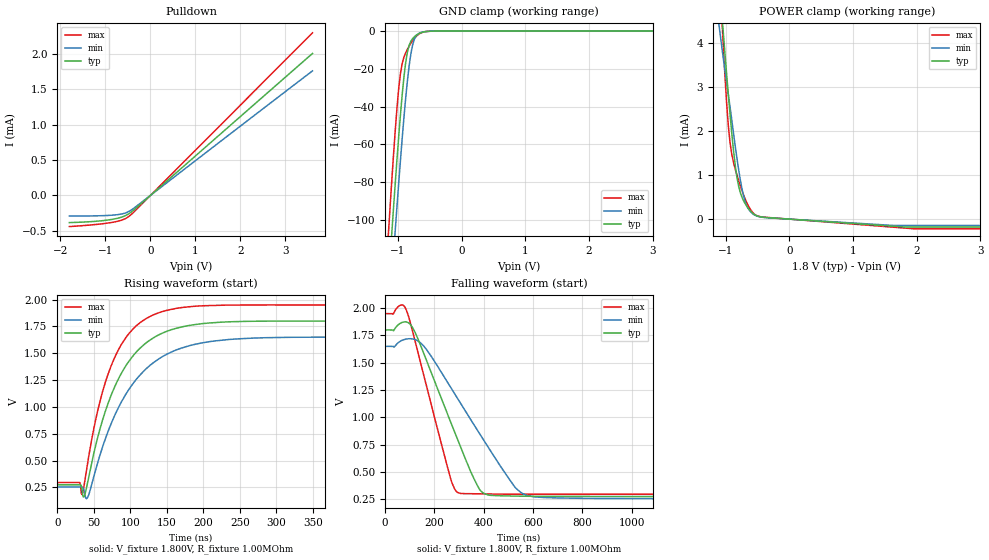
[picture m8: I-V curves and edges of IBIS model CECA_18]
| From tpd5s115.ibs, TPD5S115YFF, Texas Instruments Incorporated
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[Model]   CECA_18
Model_type   I/O_open_sink
Vinl = 800.000mV
Vinh = 2.000V
Vmeas = 1.500V
Cref = 15pF
Vref = 0V
Rref = 1000000
|   typ   min   max
|3-state
C_comp   1.1922pF   1.1689pF   1.2482pF
|pulldown
|C_comp   1.1922pF   1.1689pF   1.2481pF
[Voltage Range]   1.800V   1.650V   1.950V
|Junction temperature
[Temperature Range]   40.0   100.0   -40.0
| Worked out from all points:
|   slope of the pulldown table from 0 to 0.27 V, typ, clamps not added: 1.8 kohm
|   GND clamp passes 1 mA (typ) near -0.64 V on its own axis
|   POWER clamp passes 1 mA (typ) near -0.83 V on its own axis
|   falling waveform, V_fixture 1.800V, R_fixture 1.00MOhm: 20-80 % time 160ns typ, 234ns min, 113ns max; typ from 1.8 V to 0.274 V
|   rising waveform, V_fixture 1.800V, R_fixture 1.00MOhm: 20-80 % time 55.5ns typ, 66.4ns min, 45.9ns max; typ from 0.274 V to 1.8 V
|ambient temperature   25   85   -40|
[Pulldown]
|   Voltage   I(typ)   I(min)   I(max)
-1.8V     -382.5uA   -290uA     -439.1uA
-1.284V   -367.9uA   -288.3uA   -413.6uA
-904.5mV  -342.7uA   -280.5uA   -385.4uA
-633.2mV  -304.3uA   -260.8uA   -347.1uA
-470.4mV  -254uA     -222.9uA   -292.1uA
3.6V      2.002mA    1.756mA    2.293mA
[GND Clamp]
|   Voltage   I(typ)   I(min)   I(max)
-1.8V     -494.6mA   -503.4mA   -493.4mA
-1.149V   -134.2mA   -158mA     -107.5mA
-1.094V   -106.8mA   -131.2mA   -78.94mA
-1.04V    -80.42mA   -105.3mA   -52.46mA
-985.9mV  -55.68mA   -80.32mA   -30.36mA
-958.8mV  -44.25mA   -68.37mA   -22.43mA
-931.7mV  -33.73mA   -56.87mA   -17.18mA
-877.4mV  -16.86mA   -35.78mA   -11.65mA
-823.1mV  -7.647mA   -18.61mA   -8.038mA
-768.8mV  -4.04mA    -7.532mA   -5.134mA
-660.3mV  -1.221mA   -1.081mA   -1.428mA
3.6V      0A         0A         0A
[POWER Clamp]
|   Voltage   I(typ)   I(min)   I(max)
-1.8V     16.31mA    629.3uA    25.82mA
-1.637V   14.6mA     689.9uA    21.44mA
-1.61V    14.21mA    6.334mA    20.68mA
-1.094V   5.278mA    4.283mA    5.537mA
-1.04V    4.277mA    3.674mA    3.987mA
-958.8mV  2.821mA    2.825mA    2.114mA
-904.5mV  1.944mA    2.247mA    1.469mA
-823.1mV  944.1uA    1.373mA    995.8uA
-768.8mV  592.3uA    874.8uA    746.7uA
-687.4mV  333.7uA    370uA      432.5uA
-551.8mV  108.1uA    98.03uA    115.7uA
3.6V      -178.9uA   -145uA     -218.5uA
[Ramp]
R_load = 1.00MOhm
|   typ   min   max
dV/dt_r   915.721mV/55.535ns  837.785mV/66.415ns  993.306mV/45.899ns
dV/dt_f   915.721mV/160.192ns 837.785mV/233.633ns 993.306mV/112.781ns
[Falling Waveform]
V_fixture = 1.800V
V_fixture_min = 1.650V
V_fixture_max = 1.950V
R_fixture = 1.00MOhm
|   Time   V(typ)   V(min)   V(max)
0s        1.8V       1.65V      1.95V
66ns      1.866V     1.702V     2.029V
86ns      1.874V     1.717V     1.983V
158ns     1.578V     1.648V     1.373V
266ns     954.4mV    1.274V     432.5mV
296ns     783.9mV    1.164V     309.4mV
394ns     312.4mV    810.1mV    296.5mV
526ns     277.4mV    359.7mV    295mV
576ns     276mV      283.5mV    294.8mV
1.914us   273.8mV    253.7mV    294.5mV
[Rising Waveform]
V_fixture = 1.800V
V_fixture_min = 1.650V
V_fixture_max = 1.950V
R_fixture = 1.00MOhm
|   Time   V(typ)   V(min)   V(max)
0s        273.8mV    253.7mV    294.5mV
31ns      273.8mV    253.7mV    294.5mV
34ns      224mV      253.4mV    183mV
37ns      166.2mV    215.8mV    275.3mV
42ns      308.2mV    160.4mV    492mV
62ns      876mV      625.1mV    1.14V
94ns      1.384V     1.119V     1.647V
170ns     1.745V     1.549V     1.926V
319ns     1.8V       1.649V     1.95V
1.914us   1.8V       1.65V      1.95V
